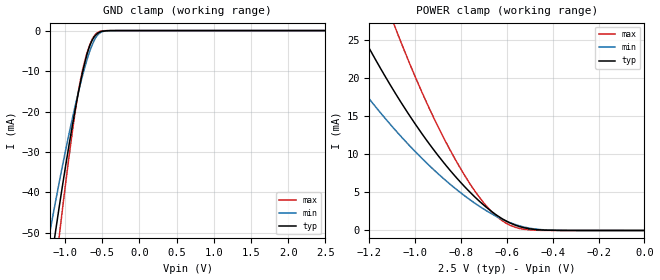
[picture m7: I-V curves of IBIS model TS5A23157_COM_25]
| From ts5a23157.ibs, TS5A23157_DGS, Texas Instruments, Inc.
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[Model]   TS5A23157_COM_25
Model_type  Terminator
| variable   typ   min   max
C_comp   16.23pF   11.39pF   18.16pF
| C_tri-state   16.23pF   11.39pF   18.16pF
[Temperature Range]   40   100   -40
| Ambient temperature   25   85   -40
[Voltage range]   2.5   2.3   2.7
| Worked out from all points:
|   GND clamp passes 1 mA (typ) near -0.58 V on its own axis
|   POWER clamp passes 1 mA (typ) near -0.59 V on its own axis
[GND Clamp]
| TS5A23157_COM_25
|   Voltage   I(typ)   I(min)   I(max)
-2.5V     -254.1mA   -206.2mA   -308.3mA
-1.205V   -59.24mA   -49.76mA   -70.99mA
-1.13V    -49.74mA   -42.33mA   -58.81mA
-1.085V   -44.21mA   -38.01mA   -51.69mA
-1.06V    -41.2mA    -35.66mA   -47.81mA
-905mV    -23.69mA   -21.89mA   -25.28mA
-790mV    -12.42mA   -12.85mA   -11.84mA
-740mV    -8.276mA   -9.375mA   -7.797mA
-670mV    -3.804mA   -5.177mA   -3.605mA
-555mV    -594.3uA   -942uA     -392.2uA
-395mV    -12.13uA   -20.23uA   -2.239uA
2.5V      2.662nA    229.9nA    2.554nA
[POWER Clamp]
| TS5A23157_COM_25
|   Voltage   I(typ)   I(min)   I(max)
-2.5V     129.7mA    93.23mA    196.3mA
-1.42V    37.04mA    26.44mA    56.81mA
-1.245V   26.36mA    18.99mA    39.91mA
-1.095V   18.41mA    13.44mA    27.23mA
-1.075V   17.43mA    12.77mA    25.68mA
-955mV    12.04mA    8.994mA    17.09mA
-835mV    7.437mA    5.749mA    9.853mA
-725mV    3.979mA    3.276mA    4.558mA
-640mV    1.915mA    1.761mA    1.734mA
-565mV    718.3uA    794.7uA    433.8uA
-475mV    123.9uA    183.6uA    35.59uA
-31.15fV  2.662nA    3.213nA    2.765nA
